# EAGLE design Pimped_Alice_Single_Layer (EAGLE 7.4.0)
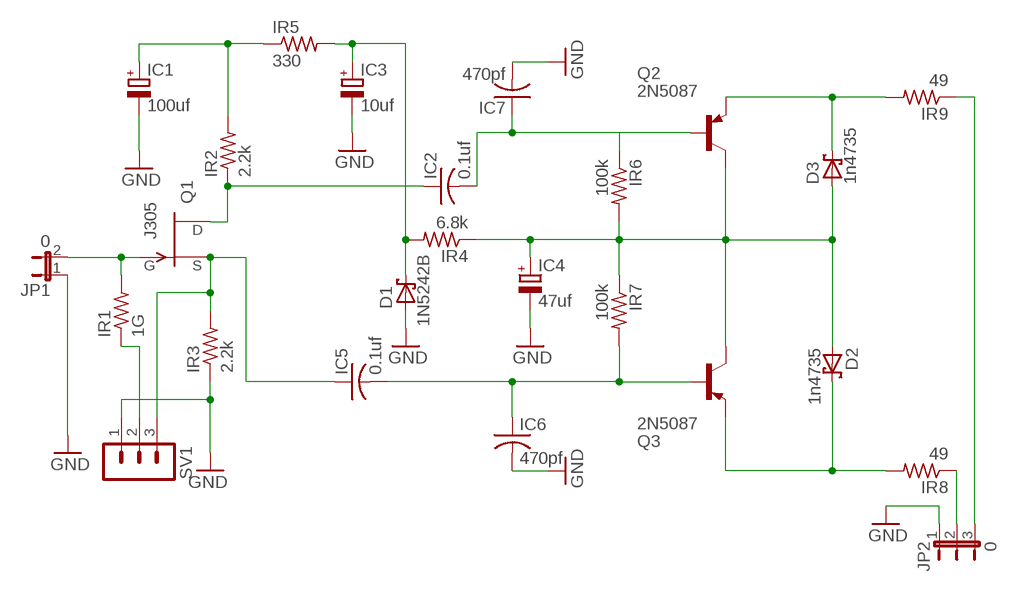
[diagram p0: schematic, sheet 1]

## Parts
D1  1N5242B  BAT42  [DO35-10]
D2  1n4735  BAT42  [DO35-10]
D3  1n4735  BAT42  [DO35-10]
IC1  100uf  CPOL-EUE2.5-7  [E2,5-7]
IC2  0.1uf  C-US050-030X075  [C050-030X075]
IC3  10uf  CPOL-EUE2.5-7  [E2,5-7]
IC4  47uf  CPOL-EUE2.5-7  [E2,5-7]
IC5  0.1uf  C-US050-030X075  [C050-030X075]
IC6  470pf  C-US050-030X075  [C050-030X075]
IC7  470pf  C-US050-030X075  [C050-030X075]
IR1  1G  R-US_0204/7  [0204/7]
IR2  2.2k  R-US_0204/7  [0204/7]
IR3  2.2k  R-US_0204/7  [0204/7]
IR4  6.8k  R-US_0204/7  [0204/7]
IR5  330  R-US_0207/2V  [0207/2V]
IR6  100k  R-US_0207/2V  [0207/2V]
IR7  100k  R-US_0207/2V  [0207/2V]
IR8  49  R-US_0207/2V  [0207/2V]
IR9  49  R-US_0207/2V  [0207/2V]
JP1  0  JP1E  [JP1]
JP2  0  JP2E  [JP2]
Q1  J305  J201  [TO92]
Q2  2N5087  2N3906  [TO92]
Q3  2N5087  2N3906  [TO92]
SV1  MA03-1  [MA03-1]

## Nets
GND: D1.A IC1.- IC3.- IC4.- IC6.2 IC7.2 IR3.1 JP1.1 JP2.1 SV1.1
N$1: IR9.1 JP2.3
N$2: IC1.+ IR2.2 IR5.1
N$3: IC2.2 IC7.1 IR6.1 Q2.2(B)
N$5: D2.C IR8.2 Q3.3(E)
N$6: D1.C IC3.+ IR4.2 IR5.2
N$7: IC2.1 IR2.1 Q1.3(D)
N$8: D2.A D3.A IC4.+ IR4.1 IR6.2 IR7.1 Q2.1(C) Q3.1(C)
N$9: IC5.2 IC6.1 IR7.2 Q3.2(B)
N$10: IC5.1 IR3.2 Q1.2(S) SV1.3
N$11: IR8.1 JP2.2
N$12: IR1.2 JP1.2 Q1.1(G)
N$13: D3.C IR9.2 Q2.3(E)
N$14: IR1.1 SV1.2

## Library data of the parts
D1-D3 = diode:BAT42: DIODE
IC1 IC3 IC4 = resistor:CPOL-EU: POLARIZED CAPACITOR, European symbol
IC2 IC5-IC7 = rcl:C-US: CAPACITOR, American symbol
IR1-IR4 = rcl:R-US_: RESISTOR, American symbol
IR5-IR9 = resistor:R-US_: RESISTOR, American symbol
JP1 = jumper:JP1E: JUMPER
JP2 = jumper:JP2E: JUMPER
Q1 = transistor-fet:?20*: TEMIC / Siliconix N-Channel JFET Source: JFET-J201_Siliconix_data.pdf
Q2 Q3 = transistor-pnp:2N3906: PNP Transistor
SV1 = con-lstb:MA03-1: PIN HEADER; OC_FARNELL: unknown; OC_NEWARK: unknown

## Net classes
0 default: width 0.635 mm, clearance 0.508 mm

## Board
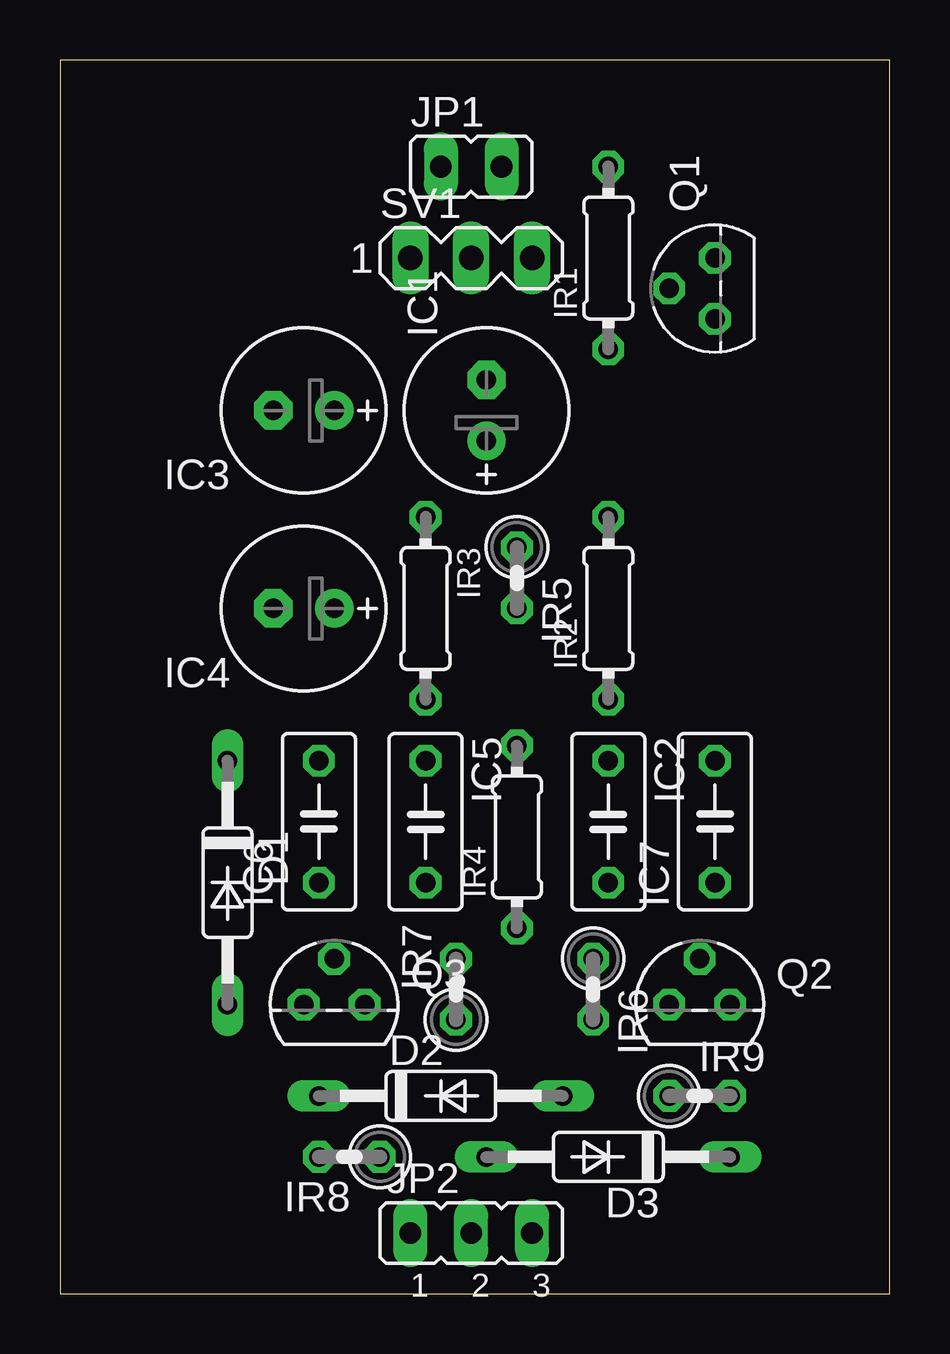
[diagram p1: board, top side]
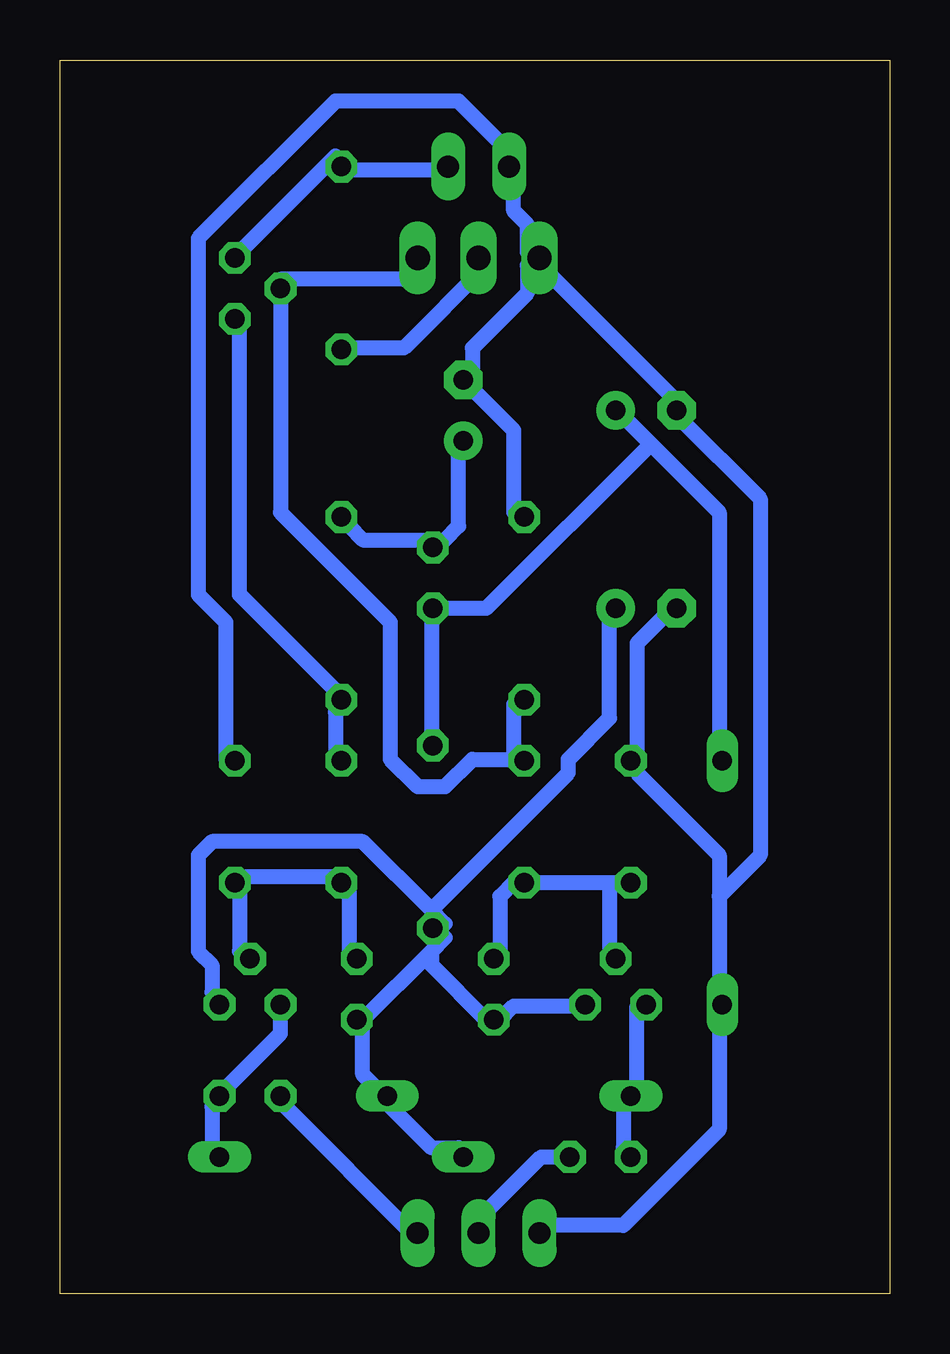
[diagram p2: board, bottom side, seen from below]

Size 34.6 x 51.44 mm. Coordinates in mm from the lower left corner, seen from the top.
Outline: 0,0 34.6,0 34.6,51.42 0.01,51.44 0,0
Copper layers (1*16): Top 0.035mm / dielectric 1.5mm / Bottom 0.035mm
Design rules "default *": minimum track width 10mil, minimum drill 24mil, track to track 15mil, track to pad 15mil, pad to pad 15mil, via to via 15mil, smd to smd 8mil, copper to edge 40mil, drill to drill 8mil, minimum pad ring 10mil, minimum via ring 8mil, stop-mask expansion 4mil, vias tented up to drill 0mil, thermal gap 10mil

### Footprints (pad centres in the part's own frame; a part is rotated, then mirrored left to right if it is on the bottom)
DO35-10 = drill 0.813 long: A 5.08,0; C -5.08,0
E2,5-7 = drill 0.813 pad 1.6: + -1.27,0 | drill 0.813 pad 1.6 octagon: - 1.27,0
C050-030X075 = drill 0.813 octagon: 1 -2.54,0; 2 2.54,0
0204/7 = drill 0.813 octagon: 1 -3.81,0; 2 3.81,0
0207/2V = drill 0.813 octagon: 1 -1.27,0; 2 1.27,0
JP1 = drill 0.914 long: 1 0,-1.27; 2 0,1.27
JP2 = drill 0.914 long: 1 -2.54,0; 2 0,0; 3 2.54,0
TO92 = drill 0.813 octagon: 1 1.27,0; 2 0,1.905; 3 -1.27,0
MA03-1 = drill 1.016 long: 1 -2.54,0; 2 0,0; 3 2.54,0

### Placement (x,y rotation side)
D1  6.98,17.15 270 top
D2  15.88,8.25 0 top
D3  22.86,5.71 180 top
IC1  17.78,36.83 90 top
IC2  22.86,19.69 270 top
IC3  10.16,36.83 180 top
IC4  10.16,28.58 180 top
IC5  15.24,19.69 270 top
IC6  10.8,19.69 90 top
IC7  27.3,19.69 90 top
IR1  22.86,43.18 90 top
IR2  22.86,28.58 90 top
IR3  15.24,28.58 270 top
IR4  19.05,19.05 90 top
IR5  19.05,29.84 270 top
IR6  22.23,12.7 270 top
IR7  16.51,12.7 90 top
IR8  12.06,5.71 180 top
IR9  26.67,8.25 0 top
JP1  17.15,46.99 270 top
JP2  17.15,2.54 0 top
Q1  27.3,41.91 90 top
Q2  26.67,12.06 0 top
Q3  11.43,12.06 0 top
SV1  17.15,43.18 0 top

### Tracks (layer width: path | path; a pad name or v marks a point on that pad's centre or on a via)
GND
  Bottom 0.635: IC4.- 9.4,28.26 10.54,27.11 10.54,22.54 IC6.2 10.54,21.72 7.11,18.29 7.11,16.57 | 7.11,16.57 7.11,12.57 D1.A 7.11,12 7.11,6.86 11.11,2.86 14.54,2.86 JP2.1 | 7.11,16.57 5.4,18.29 5.4,33.15 8.83,36.58 IC3.- 8.83,37.15 14.54,42.86 SV1.1 | SV1.1 15.11,43.43 15.11,44.58 15.68,45.15 15.68,46.86 JP1.1 15.68,47.43 17.97,49.72 23.11,49.72 28.83,44 28.83,29.15 27.69,28 27.69,22.29 IC7.2 | IR3.1 15.68,32.58 15.68,36 IC1.- 17.4,38.29 17.4,39.43 15.11,41.72 15.11,42.86 SV1.1
N$1
  Bottom 0.635: IR9.1 25.4,8 19.69,2.29 JP2.3
N$2
  Bottom 0.635: IR2.2 22.54,32 21.97,31.43 19.11,31.43 IR5.1 18.54,31.43 17.97,32 17.97,35.43 IC1.+
N$3
  Bottom 0.635: IR6.1 22.54,13.97 22.54,16.83 IC2.2 23.11,17.4 27.11,17.4 IC7.1 27.11,17.15 27.11,14.29 Q2.2
N$5
  Bottom 0.635: IR8.2 11.11,6.1 11.11,7.81 D2.C 10.54,8.57 10.54,12 Q3.3
N$6
  Bottom 0.635: 9.97,35.43 11.11,36.58 IC3.+ | 9.97,35.43 7.11,32.58 7.11,22.29 D1.C | 9.97,35.43 16.83,28.58 IR5.2 19.11,28.58 19.11,22.86 IR4.2
N$7
  Bottom 0.635: IC2.1 23.11,22.54 23.11,24.26 IR2.1 23.11,25.15 27.11,29.15 27.11,40.58 Q1.3
N$8
  Bottom 0.635: D3.A 17.97,6.1 19.11,6.1 20.83,7.81 D2.A 21.4,8.57 21.97,9.14 21.97,11.43 | 19.11,16 18.54,15.43 IR4.1 18.54,14.86 19.11,14.29 | 19.11,16 21.97,18.86 28.26,18.86 28.83,18.29 28.83,14.29 28.26,13.72 28.26,12.57 Q2.1 | 19.11,16 13.4,21.72 13.4,22.29 11.68,24 11.68,28.58 IC4.+ | Q3.1 12.83,12 15.68,12 16.26,11.43 IR7.1 16.83,11.43 19.11,13.72 19.11,14.29 | 19.11,14.29 21.97,11.43 | 21.97,11.43 IR6.2
N$9
  Bottom 0.635: 11.68,17.15 IC5.2 15.68,17.15 16.26,16.57 16.26,14.29 IR7.2 | 11.68,17.15 IC6.1 | 11.68,17.15 11.68,14.29 Q3.2
N$10
  Bottom 0.635: 15.68,22.29 15.68,24.57 IR3.2 | SV1.3 19.69,42.86 20.26,42.29 25.4,42.29 Q1.2 25.4,32.58 20.83,28 20.83,22.29 19.69,21.15 18.54,21.15 17.4,22.29 15.68,22.29 | 15.68,22.29 IC5.1
N$11
  Bottom 0.635: IR8.1 14.54,5.71 17.4,2.86 JP2.2
N$12
  Bottom 0.635: Q1.1 27.11,43.43 23.11,47.43 IR1.2 22.54,46.86 18.54,46.86 JP1.2
N$13
  Bottom 0.635: D3.C 28.26,6.1 28.26,7.81 IR9.2 27.69,8.57 25.4,10.86 Q2.3
N$14
  Bottom 0.635: IR1.1 22.54,39.43 20.26,39.43 16.83,42.86 SV1.2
